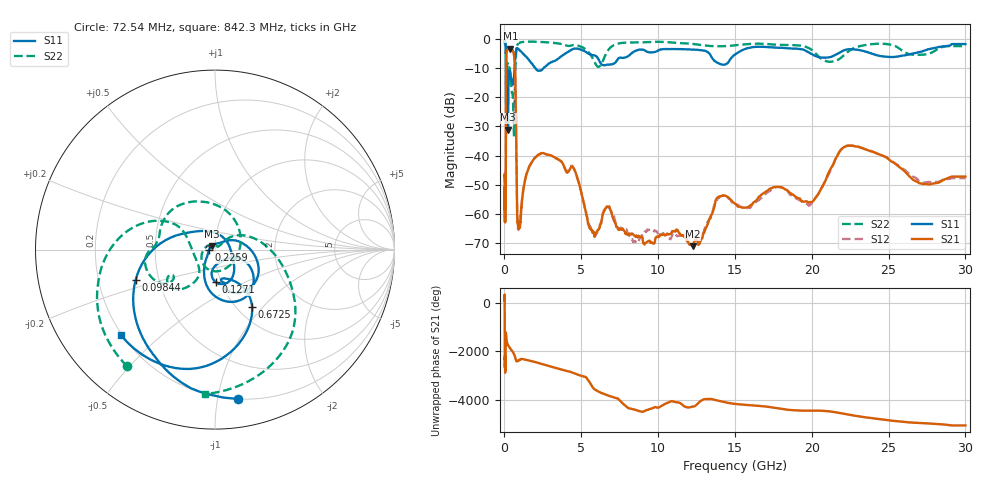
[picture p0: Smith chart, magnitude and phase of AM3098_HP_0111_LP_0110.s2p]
! Date/Time: Thu, Feb 28, 2019 8:38 AM
! Network Analyzer: Agilent Technologies E8364B Rev: A.07.50.67
! Sweep from 0.010 to 30.000 GHz, 1601 Points, Sweep Type: LOG
! Power Supply: 5.023 V, 0.002 A
# Hz S DB R 50
!freq MagS11 AngS11 MagS21 AngS21 MagS12 AngS12 MagS22 AngS22
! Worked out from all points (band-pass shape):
!   1601 points, 10 MHz to 30 GHz, reference 50 ohm
!   highest |S21| = -3.11 dB at 389.7 MHz (marker M1); lowest = -71.3 dB at 12.25 GHz (marker M2)
!   |S21| within 3 dB of the highest: 121 MHz to 640.9 MHz (520 MHz wide, 136 % of centre)
!   lowest |S11| = -31.1 dB at 231.6 MHz (marker M3), VSWR 1.06, Z = 48.1 + j1.99 ohm
!   |S11| at or under -10 dB: 102.2 MHz to 655.8 MHz (553.6 MHz wide, 146 % of centre); 2.029 GHz to 2.523 GHz (494.3 MHz wide, 21.7 % of centre)
!   |S22| runs from -33.5 to -0.5 dB; largest |S21 - S12| = 0.0096
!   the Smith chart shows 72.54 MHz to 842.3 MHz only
!   S11 on the Smith chart (normalised r, x): 72.54 MHz: 0.20, -1.15; 98.44 MHz: 0.37, -0.16; 127.1 MHz: 0.94, -0.35; 225.9 MHz: 0.94, -0.00; 672.5 MHz: 1.17, -0.88; 842.3 MHz: 0.20, -0.37
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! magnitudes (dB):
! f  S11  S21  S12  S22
! 10 MHz  -0.3  -47.2  -45.8  -0.5
! 38.04 MHz  -0.4  -58.7  -60.1  -0.8
! 72.54 MHz  -1.5  -52.4  -53.0  -1.8
! 84.29 MHz  -2.4  -56.1  -53.0  -2.6
! 98.44 MHz  -6.5  -27.4  -27.4  -7.3
! 127.1 MHz  -14.8  -5.4  -5.4  -9.8
! 144.7 MHz  -20.1  -4.2  -4.1  -11.2
! 183.1 MHz  -10.5  -3.8  -3.7  -8.0
! 225.9 MHz  -29.5  -3.3  -3.3  -9.4
! 231.6 MHz  -31.1  -3.2  -3.2  -9.5
! 389.7 MHz  -11.8  -3.1  -3.1  -12.0
! 550.5 MHz  -15.6  -3.9  -3.9  -20.5
! 620.7 MHz  -13.2  -5.3  -5.2  -33.4
! 672.5 MHz  -8.4  -8.3  -8.3  -19.4
! 842.3 MHz  -3.0  -61.7  -61.8  -1.9
! 2.084 GHz  -10.4  -40.3  -40.3  -0.8
! 4.436 GHz  -3.3  -43.9  -43.7  -1.9
! 7.926 GHz  -6.1  -66.6  -65.4  -1.1
! 12.25 GHz  -3.5  -71.3  -68.1  -1.5
! 19.8 GHz  -4.5  -56.3  -57.3  -3.0
! 22.56 GHz  -3.4  -36.6  -36.5  -3.5
! 30 GHz  -1.6  -47.3  -47.8  -2.3
